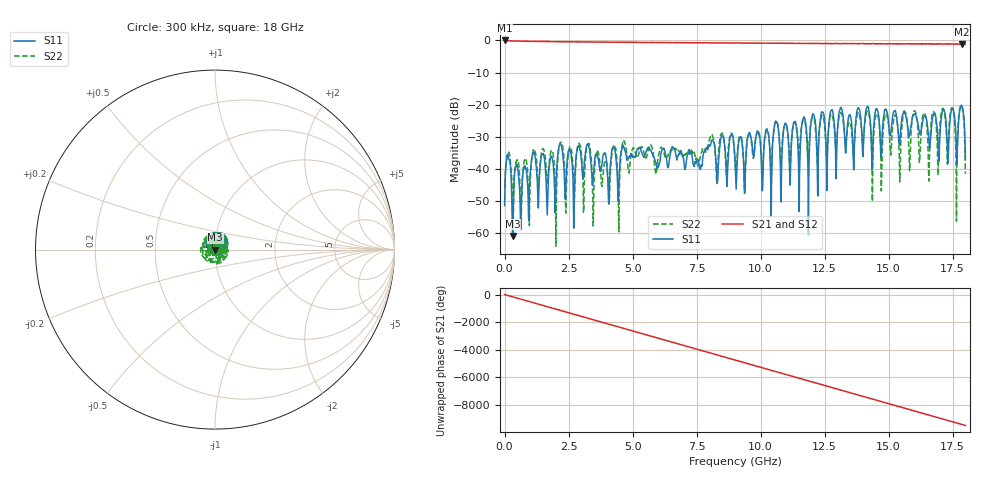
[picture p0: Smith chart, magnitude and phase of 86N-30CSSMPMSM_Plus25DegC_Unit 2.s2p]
!Agilent Technologies,N5230A,MY45000342,A.06.04.32
!Agilent N5230A: A.06.04.32
!Date: Thursday, March 12, 2026 14:21:48
!Correction: S11(Full 2 Port(1,4)) S41(Full 2 Port(1,4)) S14(Full 2 Port(1,4)) S44(Full 2 Port(1,4))
!S2P File: Measurements: S11, S41, S14, S44:
# Hz S  dB  R 50
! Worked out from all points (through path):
!   1601 points, 300 kHz to 18 GHz, reference 50 ohm
!   highest |S21| = 0.00 dB at 300 kHz (marker M1); lowest = -1.2 dB at 17.87 GHz (marker M2)
!   group delay of S21, straight-line fit = 1.46 ns
!   lowest |S11| = -60.8 dB at 315.3 MHz (marker M3), VSWR 1.00, Z = 50.1 + j0.0168 ohm
!   |S11| at or under -10 dB: start of sweep to end of sweep
!   |S22| runs from -64.0 to -20.2 dB; largest |S21 - S12| = 0.017
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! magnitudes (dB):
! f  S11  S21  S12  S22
! 300 kHz  -51.3  0.0  0.0  -44.4
! 146.5 MHz  -36.4  -0.1  -0.2  -35.1
! 315.3 MHz  -60.8  -0.2  -0.2  -52.0
! 1.125 GHz  -35.0  -0.3  -0.3  -33.9
! 3.004 GHz  -37.5  -0.5  -0.5  -35.6
! 6.008 GHz  -39.2  -0.6  -0.7  -35.8
! 9 GHz  -36.8  -0.8  -0.9  -38.2
! 10.25 GHz  -27.7  -0.9  -0.9  -27.5
! 10.42 GHz  -52.7  -0.9  -0.9  -43.6
! 10.61 GHz  -25.2  -0.9  -0.9  -25.0
! 10.79 GHz  -49.9  -0.9  -0.9  -37.7
! 11.33 GHz  -25.3  -0.9  -1.0  -25.4
! 11.51 GHz  -53.2  -0.9  -0.9  -36.6
! 11.69 GHz  -23.9  -0.9  -1.0  -24.6
! 11.87 GHz  -60.5  -0.9  -0.9  -37.6
! 12 GHz  -23.9  -1.0  -1.0  -24.2
! 12.23 GHz  -48.2  -0.9  -1.0  -37.3
! 15.01 GHz  -26.6  -1.0  -1.0  -26.7
! 17.48 GHz  -21.1  -1.1  -1.2  -20.9
! 17.65 GHz  -36.5  -1.2  -1.2  -56.2
! 17.87 GHz  -20.4  -1.2  -1.3  -20.7
! 18 GHz  -36.9  -1.1  -1.2  -41.5
